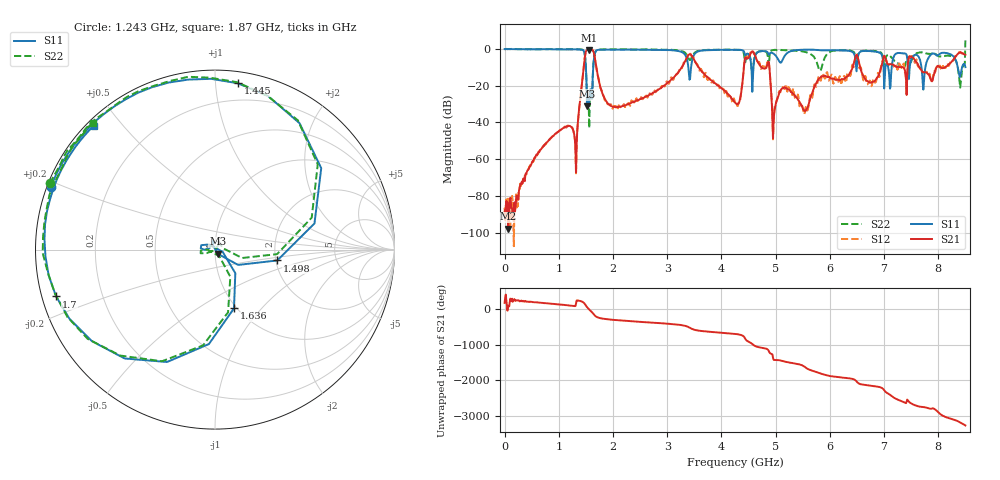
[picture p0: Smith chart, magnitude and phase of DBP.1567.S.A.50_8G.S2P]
!iTest VNA485 VNA485-80111 1.8.6.282
!Date: Wed Mar 20 17:05:34 2024
!Data & Calibration Information:
!Freq	S11:SOLT2(ON)	S21:SOLT2(ON)	S12:SOLT2(ON)	S22:SOLT2(ON)
!PortZ  Port1:50+j0  Port2:50+j0
!Above PortZ is port z conversion or system Z0 setting when saving the data.
!When reading, reference impedance value at option line is always used.
# Hz S RI R 50
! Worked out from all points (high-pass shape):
!   801 points, 300 kHz to 8.5 GHz, reference 50 ohm
!   highest |S21| = -0.45 dB at 1.562 GHz (marker M1); lowest = -97.9 dB at 64.05 MHz (marker M2)
!   |S21| within 3 dB of the highest: 1.485 GHz to 1.656 GHz (171 MHz wide, 10.9 % of centre); 8.337 GHz to end of sweep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
!   lowest |S11| = -31.2 dB at 1.52 GHz (marker M3), VSWR 1.06, Z = 51.5 - j2.38 ohm
!   |S11| at or under -10 dB: 1.5 GHz to 1.635 GHz (135.4 MHz wide, 8.64 % of centre); 7.689 GHz to 7.762 GHz (73.16 MHz wide, 0.947 % of centre); 8.359 GHz to 8.438 GHz (78.72 MHz wide, 0.937 % of centre)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
!   |S22| runs from -43.1 to 4.7 dB; largest |S21 - S12| = 0.12
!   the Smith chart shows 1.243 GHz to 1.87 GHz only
!   S11 on the Smith chart (normalised r, x): 1.243 GHz: 0.01, +0.18; 1.445 GHz: 0.08, +1.14; 1.498 GHz: 2.04, -0.28; 1.636 GHz: 0.97, -0.72; 1.7 GHz: 0.04, -0.14; 1.87 GHz: 0.02, +0.42
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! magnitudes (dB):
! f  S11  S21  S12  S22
! 300 kHz  0.0  -88.9  -86.5  0.0
! 64.05 MHz  0.0  -97.9  -81.5  0.0
! 1.243 GHz  -0.2  -43.0  -42.6  -0.1
! 1.328 GHz  -0.2  -52.6  -52.7  -0.1
! 1.424 GHz  -0.4  -19.7  -19.9  -0.2
! 1.445 GHz  -0.6  -13.9  -14.2  -0.5
! 1.498 GHz  -9.1  -1.4  -1.6  -9.2
! 1.52 GHz  -31.2  -0.6  -0.6  -26.9
! 1.562 GHz  -30.0  -0.5  -0.4  -43.1
! 1.636 GHz  -9.3  -1.2  -1.4  -8.9
! 1.7 GHz  -0.7  -11.3  -11.9  -0.7
! 1.87 GHz  -0.3  -28.2  -27.6  -0.2
! 2.837 GHz  -0.5  -22.0  -21.6  -0.3
! 3.411 GHz  -16.7  -2.8  -2.9  -5.9
! 4.25 GHz  -0.4  -29.2  -29.8  -0.3
! 4.569 GHz  -23.3  -1.2  -1.2  -16.5
! 4.856 GHz  -2.0  -7.7  -6.4  -4.1
! 4.973 GHz  -2.8  -35.2  -34.9  -0.6
! 5.674 GHz  -0.3  -23.9  -26.5  -3.3
! 7.087 GHz  -11.9  -8.4  -8.8  -3.2
! 8.404 GHz  -14.8  -1.8  -1.6  -21.0
! 8.5 GHz  -9.8  -3.1  -3.0  4.7
